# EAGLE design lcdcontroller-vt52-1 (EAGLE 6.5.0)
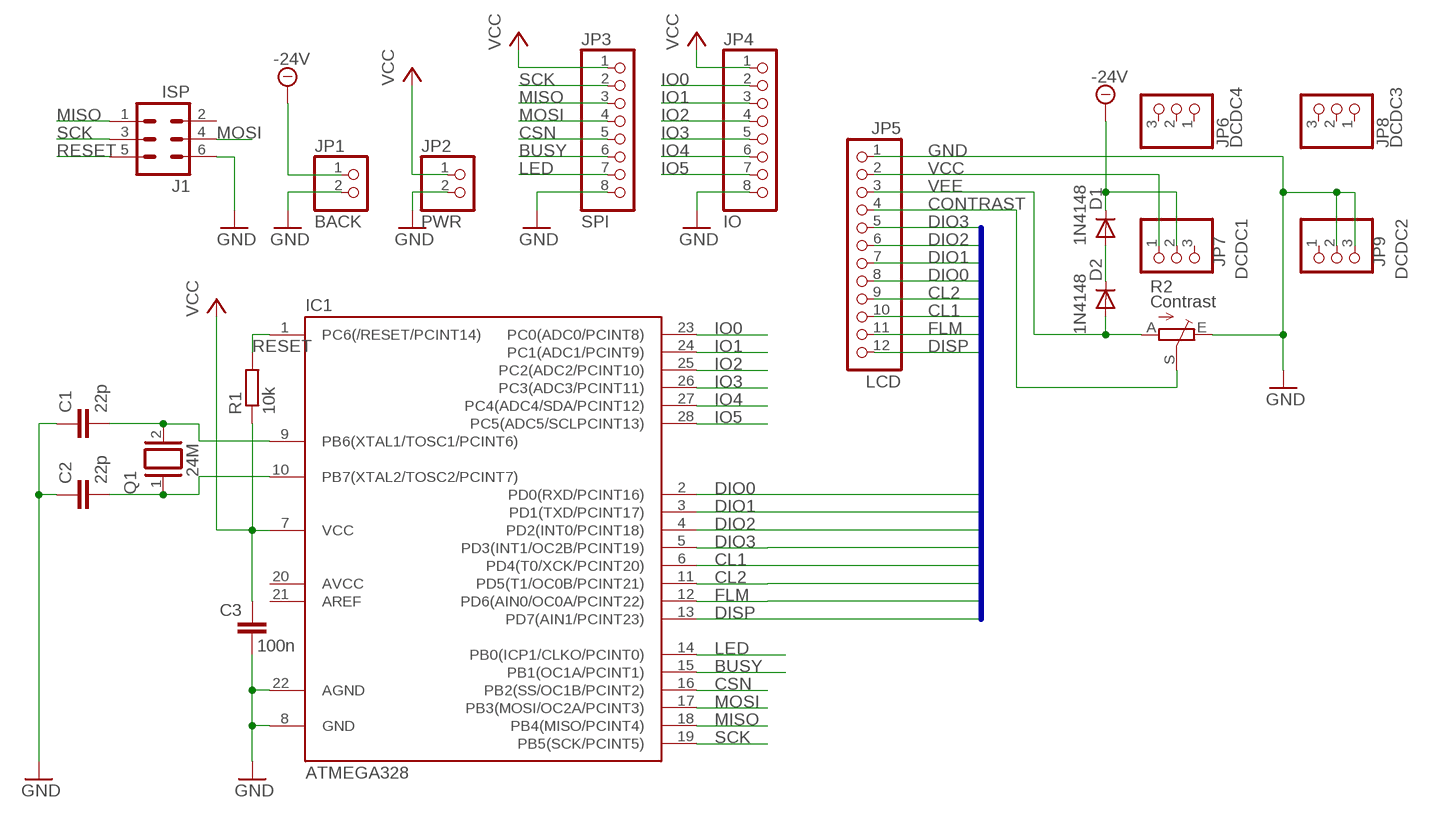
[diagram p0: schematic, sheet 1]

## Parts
C1  22p  C-EU025-024X044  [C025-024X044]
C2  22p  C-EU025-024X044  [C025-024X044]
C3  100n  C-EU025-024X044  [C025-024X044]
D1  1N4148  1N4148DO35-7  [DO35-7]
D2  1N4148  1N4148DO35-7  [DO35-7]
IC1  ATMEGA328  MEGA48/88/168-PU  [DIL28-3]
J1  ISP  ML6  [ML6]
JP1  BACK  PINHD-1X2  [1X02]
JP2  PWR  PINHD-1X2  [1X02]
JP3  SPI  PINHD-1X8  [1X08]
JP4  IO  PINHD-1X8  [1X08]
JP5  LCD  PINHD-1X12  [1X12]
JP6  DCDC4  PINHD-1X3  [1X03]
JP7  DCDC1  PINHD-1X3  [1X03]
JP8  DCDC3  PINHD-1X3  [1X03]
JP9  DCDC2  PINHD-1X3  [1X03]
Q1  24M  XTAL/S  [QS]
R1  10k  R-EU_0207/10  [0207/10]
R2  Contrast  TRIM_EU-PT10S  [PT-10S]

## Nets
-24V: D1.C JP1.1 JP7.2
BUSY: IC1.15(PB1(OC1A/PCINT1)) JP3.6
CL1: IC1.6(PD4(T0/XCK/PCINT20)) JP5.10
CL2: IC1.11(PD5(T1/OC0B/PCINT21)) JP5.9
CONTRAST: JP5.4 R2.S
CSN: IC1.16(PB2(SS/OC1B/PCINT2)) JP3.5
DIO0: IC1.2(PD0(RXD/PCINT16)) JP5.8
DIO1: IC1.3(PD1(TXD/PCINT17)) JP5.7
DIO2: IC1.4(PD2(INT0/PCINT18)) JP5.6
DIO3: IC1.5(PD3(INT1/OC2B/PCINT19)) JP5.5
DISP: IC1.13(PD7(AIN1/PCINT23)) JP5.12
FLM: IC1.12(PD6(AIN0/OC0A/PCINT22)) JP5.11
GND: C1.1 C2.1 C3.1 IC1.8(GND) IC1.22(AGND) J1.6 JP1.2 JP2.2 JP3.8 JP4.8 JP5.1 JP9.2 JP9.3 R2.E
IO0: IC1.23(PC0(ADC0/PCINT8)) JP4.2
IO1: IC1.24(PC1(ADC1/PCINT9)) JP4.3
IO2: IC1.25(PC2(ADC2/PCINT10)) JP4.4
IO3: IC1.26(PC3(ADC3/PCINT11)) JP4.5
IO4: IC1.27(PC4(ADC4/SDA/PCINT12)) JP4.6
IO5: IC1.28(PC5(ADC5/SCLPCINT13)) JP4.7
LED: IC1.14(PB0(ICP1/CLKO/PCINT0)) JP3.7
MISO: IC1.18(PB4(MISO/PCINT4)) J1.1 JP3.3
MOSI: IC1.17(PB3(MOSI/OC2A/PCINT3)) J1.4 JP3.4
N$9: D1.A D2.C
RESET: IC1.1(PC6(/RESET/PCINT14)) J1.5 R1.2
SCK: IC1.19(PB5(SCK/PCINT5)) J1.3 JP3.2
VCC: C3.2 IC1.7(VCC) JP2.1 JP3.1 JP4.1 JP5.2 JP7.1 R1.1
VEE: D2.A JP5.3 R2.A
XTAL1: C1.2 IC1.9(PB6(XTAL1/TOSC1/PCINT6)) Q1.2
XTAL2: C2.2 IC1.10(PB7(XTAL2/TOSC2/PCINT7)) Q1.1
Unconnected: IC1.20(AVCC) IC1.21(AREF) J1.2 JP6.1 JP6.2 JP6.3 JP7.3 JP8.1 JP8.2 JP8.3 JP9.1

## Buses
BUS:DIO[0..3],FLM,CL1,CL2,DISP

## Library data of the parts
C1-C3 = rcl:C-EU: CAPACITOR, European symbol
D1 D2 = diode:1N4148: DIODE
IC1 = avr-7:MEGA48/88/168-PU
J1 = con-harting-ml:ML6: HARTING; OC_FARNELL: unknown; OC_NEWARK: unknown
JP1 JP2 = pinhead:PINHD-1X2: PIN HEADER
JP3 JP4 = pinhead:PINHD-1X8: PIN HEADER
JP5 = pinhead:PINHD-1X12: PIN HEADER
JP6-JP9 = pinhead:PINHD-1X3: PIN HEADER
Q1 = special:XTAL/S: CRYSTAL
R1 = rcl:R-EU_: RESISTOR, European symbol
R2 = pot:TRIM_EU-: POTENTIOMETER

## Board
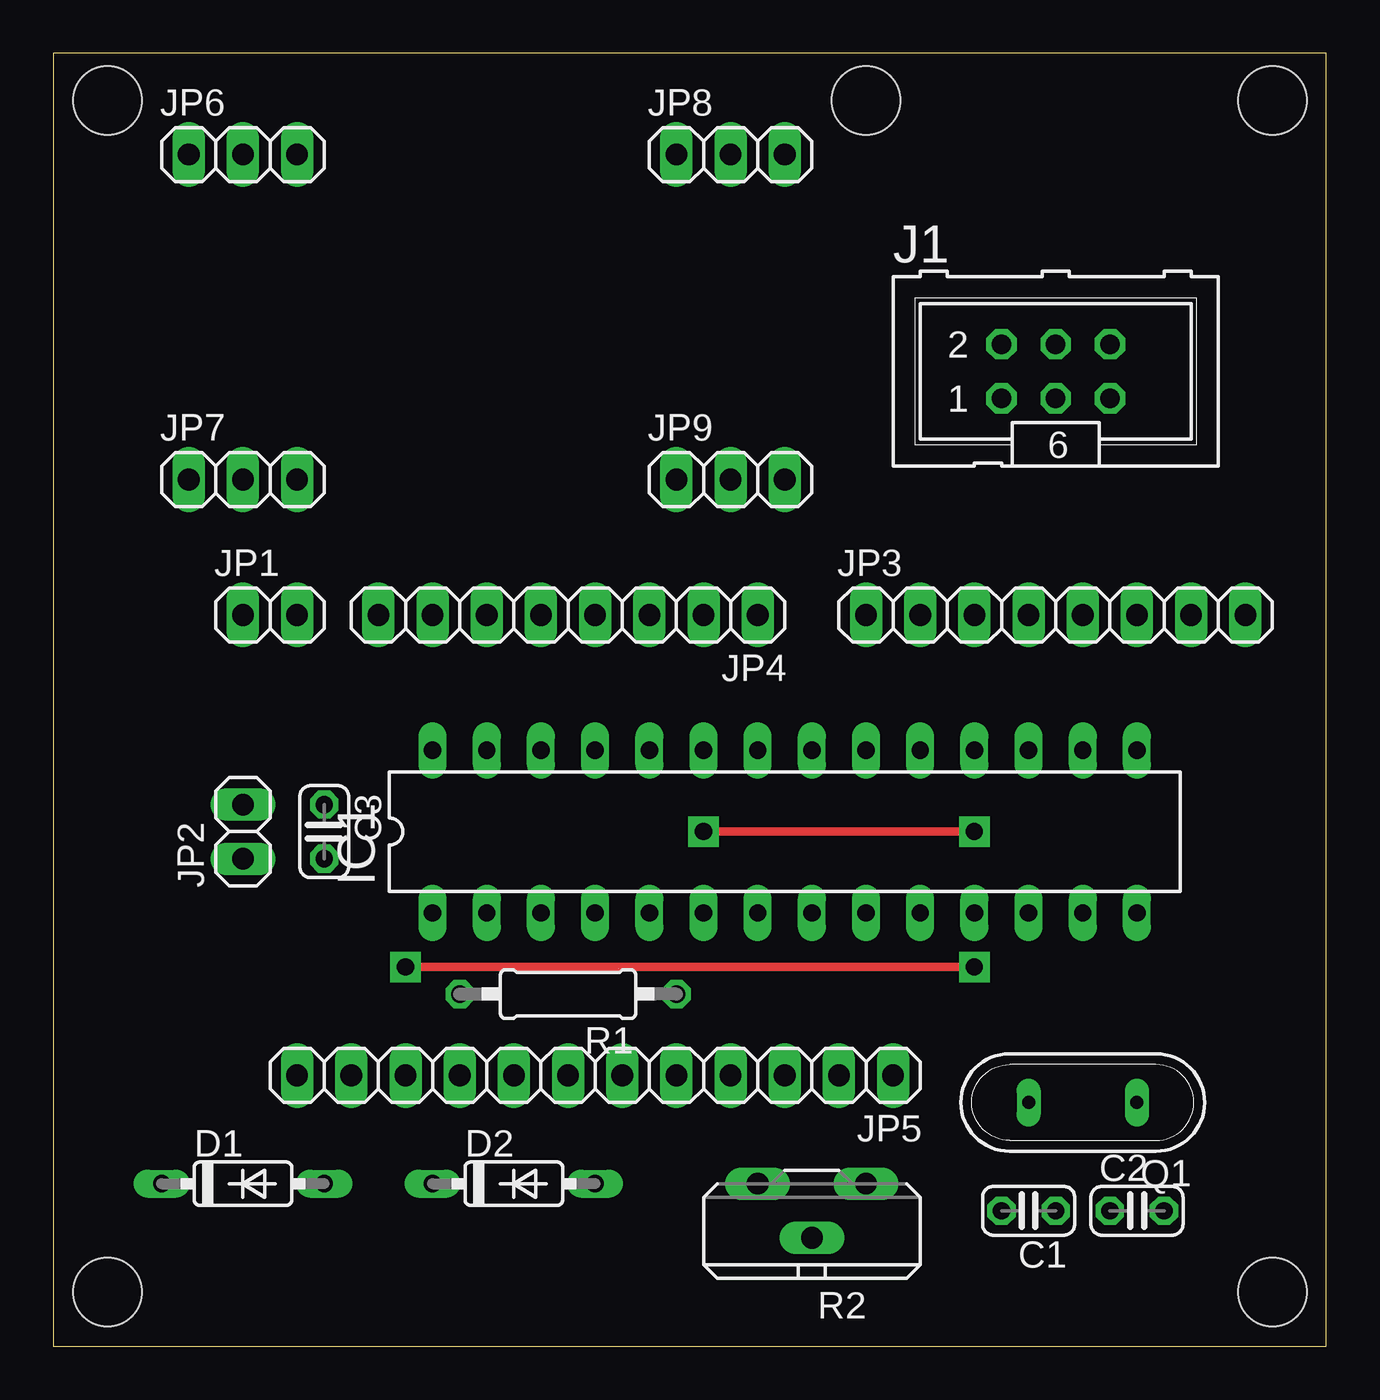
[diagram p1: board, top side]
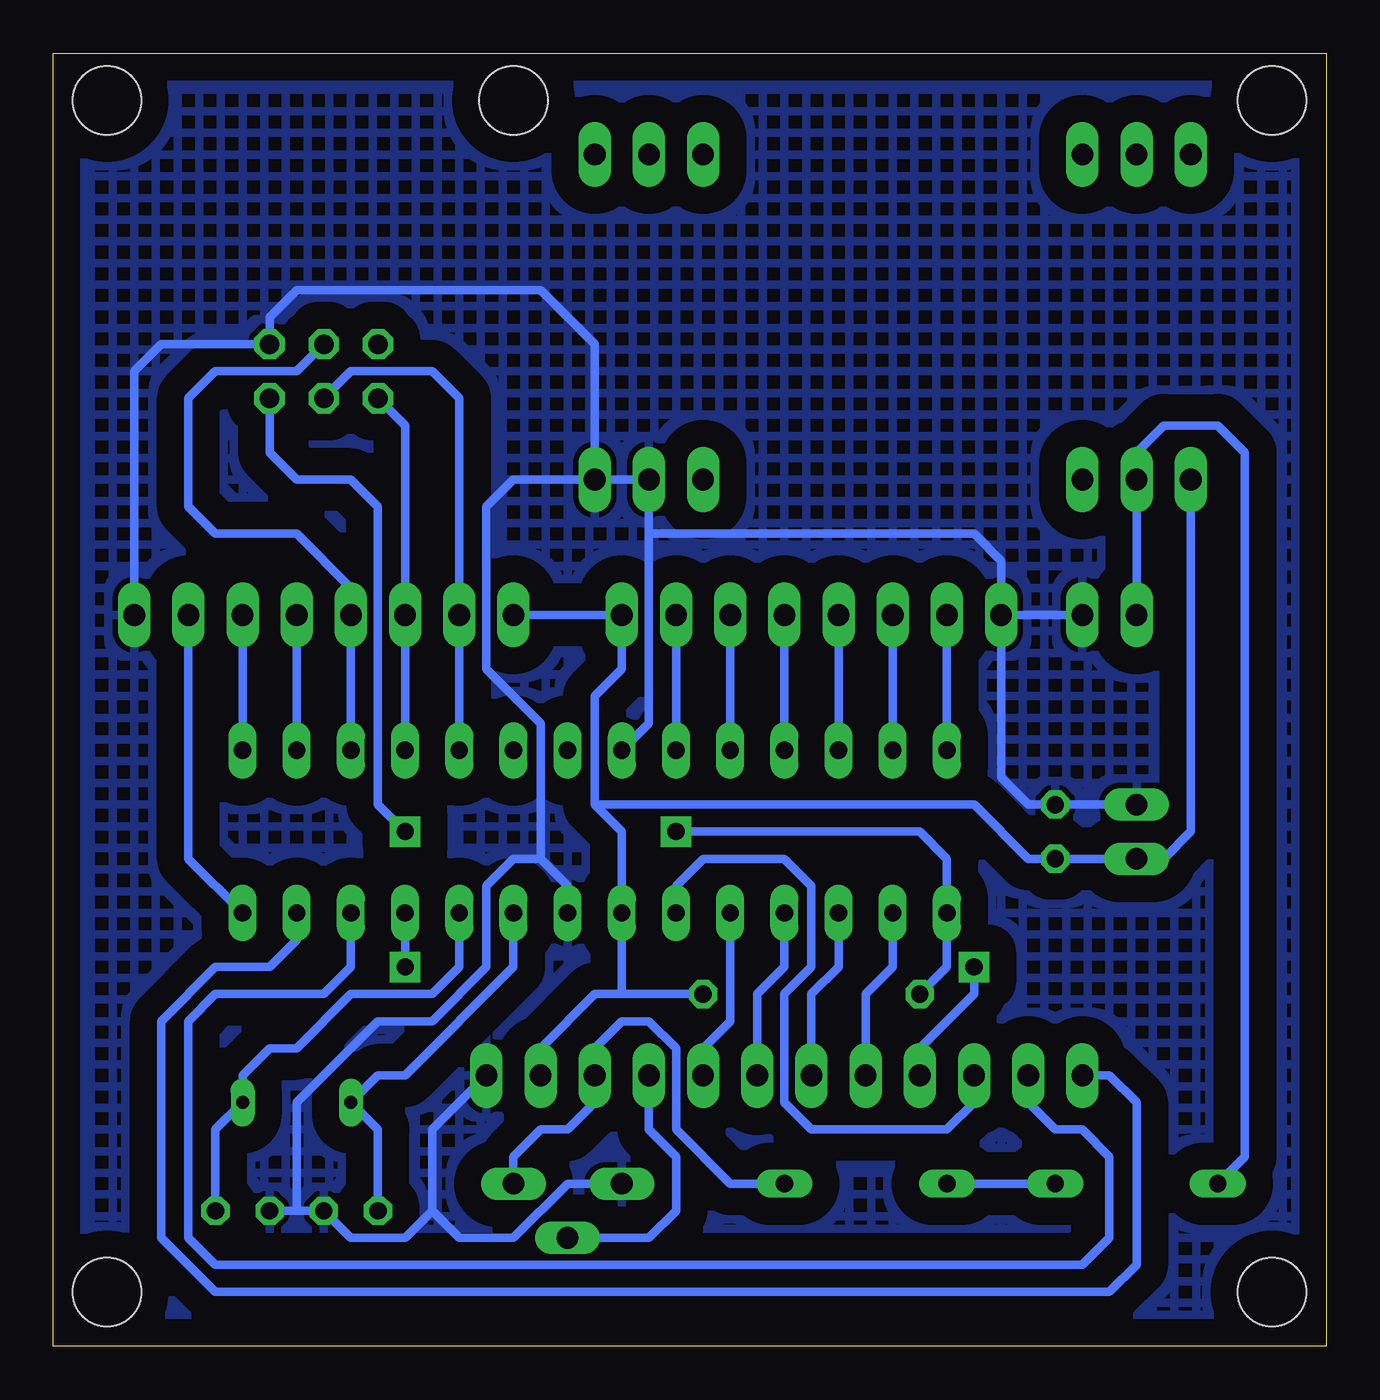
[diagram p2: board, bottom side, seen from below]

Size 59.67 x 60.63 mm. Coordinates in mm from the lower left corner, seen from the top.
Outline: 0,0 59.67,0 59.67,60.63 0,60.63 0,0
Copper layers (1*16): Top 0.035mm / dielectric 1.5mm / Bottom 0.035mm
Design rules "default": minimum track width 10mil, minimum drill 24mil, track to track 8mil, track to pad 8mil, pad to pad 8mil, via to via 8mil, smd to smd 8mil, copper to edge 40mil, drill to drill 8mil, minimum pad ring 10mil, minimum via ring 8mil, stop-mask expansion 4mil, vias tented up to drill 0mil, thermal gap 10mil
Holes 3.2 mm at 2.54,2.54 57.15,2.54 57.15,58.42 2.54,58.42 38.1,58.42

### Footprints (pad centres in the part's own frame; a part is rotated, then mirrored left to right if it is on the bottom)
C025-024X044 = drill 0.813 octagon: 1 -1.27,0; 2 1.27,0
DO35-7 = drill 0.813 long: A 3.81,0; C -3.81,0
DIL28-3 = drill 0.813 long: 1 -16.51,-3.81; 2 -13.97,-3.81; 3 -11.43,-3.81; 4 -8.89,-3.81; 5 -6.35,-3.81; 6 -3.81,-3.81; 7 -1.27,-3.81; 8 1.27,-3.81; 9 3.81,-3.81; 10 6.35,-3.81; 11 8.89,-3.81; 12 11.43,-3.81; 13 13.97,-3.81; 14 16.51,-3.81; 15 16.51,3.81; 16 13.97,3.81; 17 11.43,3.81; 18 8.89,3.81; 19 6.35,3.81; 20 3.81,3.81; 21 1.27,3.81; 22 -1.27,3.81; 23 -3.81,3.81; 24 -6.35,3.81; 25 -8.89,3.81; 26 -11.43,3.81; 27 -13.97,3.81; 28 -16.51,3.81
ML6 = drill 0.914 octagon: 1 -2.54,-1.27; 2 -2.54,1.27; 3 0,-1.27; 4 0,1.27; 5 2.54,-1.27; 6 2.54,1.27
1X02 = drill 1.016 long: 1 -1.27,0; 2 1.27,0
1X08 = drill 1.016 long: 1 -8.89,0; 2 -6.35,0; 3 -3.81,0; 4 -1.27,0; 5 1.27,0; 6 3.81,0; 7 6.35,0; 8 8.89,0
1X12 = drill 1.016 long: 1 -13.97,0; 2 -11.43,0; 3 -8.89,0; 4 -6.35,0; 5 -3.81,0; 6 -1.27,0; 7 1.27,0; 8 3.81,0; 9 6.35,0; 10 8.89,0; 11 11.43,0; 12 13.97,0
1X03 = drill 1.016 long: 1 -2.54,0; 2 0,0; 3 2.54,0
QS = drill 0.61 long: 1 -2.54,0; 2 2.54,0
0207/10 = drill 0.813 octagon: 1 -5.08,0; 2 5.08,0
PT-10S = drill 1.016 long: A -2.54,-1.27; E 2.54,-1.27; S 0,1.27

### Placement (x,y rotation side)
C1  45.72,6.35 180 top
C2  50.8,6.35 0 top
C3  12.7,24.13 270 top
D1  8.89,7.62 0 top
D2  21.59,7.62 0 top
IC1  34.29,24.13 0 top
J1  46.99,45.72 0 top
JP1  10.16,34.29 0 top
JP2  8.89,24.13 90 top
JP3  46.99,34.29 0 top
JP4  24.13,34.29 180 top
JP5  25.4,12.7 180 top
JP6  8.89,55.88 0 top
JP7  8.89,40.64 0 top
JP8  31.75,55.88 0 top
JP9  31.75,40.64 0 top
Q1  48.26,11.43 180 top
R1  24.13,16.51 180 top
R2  35.56,6.35 180 top

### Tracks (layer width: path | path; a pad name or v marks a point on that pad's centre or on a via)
-24V
  Bottom 0.406: JP1.1 JP7.2 8.89,41.91 7.62,43.18 5.08,43.18 3.81,41.91 3.81,8.89 D1.C
BUSY
  Bottom 0.406: JP3.6 IC1.15
CL1
  Bottom 0.406: JP5.10 16.51,11.43 17.78,10.16 24.13,10.16 25.4,11.43 25.4,16.51 24.13,17.78 24.13,21.59 25.4,22.86 29.21,22.86 30.48,21.59 IC1.6
CL2  (via drill 0.8 pad 1.42)
  Top 0.406: v16.51,17.78 v43.18,17.78
  Bottom 0.406: JP5.9 19.05,13.97 16.51,16.51 v16.51,17.78 | v43.18,17.78 IC1.11
CONTRAST
  Bottom 0.406: R2.S 31.75,5.08 30.48,6.35 30.48,8.89 31.75,10.16 JP5.4
CSN
  Bottom 0.406: JP3.5 IC1.16
DIO0
  Bottom 0.406: IC1.2 20.32,17.78 21.59,16.51 JP5.8
DIO1
  Bottom 0.406: IC1.3 22.86,17.78 24.13,16.51 JP5.7
DIO2
  Bottom 0.406: IC1.4 25.4,17.78 26.67,16.51 JP5.6
DIO3
  Bottom 0.406: IC1.5 27.94,15.24 29.21,13.97 JP5.5
DISP
  Bottom 0.406: JP5.12 10.16,12.7 8.89,11.43 8.89,3.81 10.16,2.54 52.07,2.54 54.61,5.08 54.61,15.24 52.07,17.78 49.53,17.78 48.26,19.05 IC1.13
FLM
  Bottom 0.406: JP5.11 13.97,11.43 12.7,10.16 11.43,10.16 10.16,8.89 10.16,5.08 11.43,3.81 52.07,3.81 53.34,5.08 53.34,15.24 52.07,16.51 46.99,16.51 45.72,17.78 IC1.12
GND
  Bottom 0.406: JP1.2 JP4.8 | JP4.8 15.24,36.83 16.51,38.1 31.75,38.1 | 31.75,38.1 JP9.2 JP9.3 | JP2.2 C3.1 13.97,25.4 15.24,26.67 JP4.8 | JP9.3 34.29,46.99 36.83,49.53 48.26,49.53 49.53,48.26 J1.6 54.61,46.99 55.88,45.72 JP3.8 | R2.E 35.56,7.62 38.1,5.08 40.64,5.08 41.91,6.35 | 41.91,6.35 41.91,10.16 JP5.1 | C2.1 48.26,6.35 | 48.26,6.35 C1.1 45.72,5.08 43.18,5.08 41.91,6.35 | 48.26,6.35 48.26,11.43 44.45,15.24 41.91,15.24 39.37,17.78 39.37,21.59 38.1,22.86 36.83,22.86 | 36.83,22.86 35.56,21.59 IC1.8 | 36.83,22.86 36.83,29.21 39.37,31.75 39.37,39.37 38.1,40.64 JP9.3 | 31.75,38.1 31.75,29.21 IC1.22
  pour Bottom (isolate 1.27, hatched): 0,60.96 59.69,60.96 59.69,0 0,0
IO0
  Bottom 0.406: JP4.2 IC1.23
IO1
  Bottom 0.406: JP4.3 IC1.24
IO2
  Bottom 0.406: JP4.4 IC1.25
IO3
  Bottom 0.406: JP4.5 IC1.26
IO4
  Bottom 0.406: JP4.6 IC1.27
IO5
  Bottom 0.406: JP4.7 IC1.28
LED
  Bottom 0.406: IC1.14 53.34,22.86 JP3.7
MISO
  Bottom 0.406: IC1.18 JP3.3 43.18,43.18 J1.1
MOSI
  Bottom 0.406: IC1.17 JP3.4 45.72,35.56 48.26,38.1 52.07,38.1 53.34,39.37 53.34,44.45 52.07,45.72 48.26,45.72 J1.4
N$9
  Bottom 0.406: D1.A D2.C
RESET  (via drill 0.8 pad 1.42)
  Top 0.406: v30.48,24.13 v43.18,24.13
  Bottom 0.406: R1.2 17.78,17.78 IC1.1 17.78,22.86 19.05,24.13 v30.48,24.13 | v43.18,24.13 44.45,25.4 44.45,39.37 45.72,40.64 48.26,40.64 49.53,41.91 J1.5
SCK
  Bottom 0.406: IC1.19 JP3.2 40.64,44.45 41.91,45.72 45.72,45.72 J1.3
VCC
  Bottom 0.406: JP3.1 JP4.1 33.02,31.75 34.29,30.48 34.29,25.4 | JP7.1 6.35,24.13 7.62,22.86 JP2.1 C3.2 13.97,22.86 16.51,25.4 34.29,25.4 | 33.02,16.51 IC1.7 33.02,24.13 34.29,25.4 | 33.02,16.51 R1.1 | JP5.2 36.83,13.97 34.29,16.51 33.02,16.51
VEE
  Bottom 0.406: R2.A 38.1,8.89 36.83,10.16 35.56,10.16 34.29,11.43 JP5.3 34.29,13.97 33.02,15.24 31.75,15.24 30.48,13.97 30.48,10.16 27.94,7.62 D2.A
XTAL1
  Bottom 0.406: C1.2 44.45,10.16 Q1.2 44.45,12.7 43.18,12.7 38.1,17.78 IC1.9
XTAL2
  Bottom 0.406: C2.2 52.07,10.16 Q1.1 50.8,12.7 49.53,13.97 48.26,13.97 45.72,16.51 41.91,16.51 40.64,17.78 IC1.10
